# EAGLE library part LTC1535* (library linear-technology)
Isolated RS485 Transceiver Source : www.linear.com
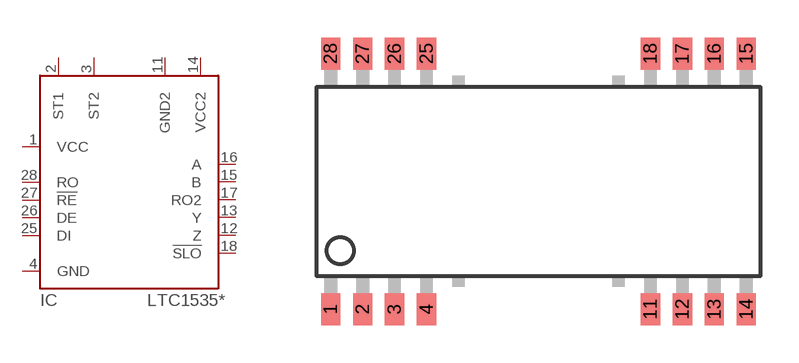
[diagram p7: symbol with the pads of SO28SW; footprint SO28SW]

Designator prefix IC

## LTC1535CSW (MPN: LTC1535CSW; OC_FARNELL: 1609802; OC_NEWARK: 56M1820), LTC1535ISW (MPN: LTC1535ISW; OC_FARNELL: 1498465; OC_NEWARK: 56M1824)  [SO28SW]
1  VCC  in
2  ST1  in
3  ST2  in
4  GND  in
11  GND2  in
12  Z  hiz
13  Y  hiz
14  VCC2  in
15  B  in
16  A  in
17  RO2  out
18  !SLO  in
25  DI  in
26  DE  in
27  !RE  in
28  RO  out

## Footprint SO28SW (pad centres in mm)
28-Lead Plastic Small Outline Isolation Barrier (Wide .300 Inch) Reference LTC DWG # 05-08-1690 Source: www.linear.com
smd 0.762 x 1.27: 1 -8.255,-5.08; 2 -6.985,-5.08; 3 -5.715,-5.08; 4 -4.445,-5.08; 11 4.445,-5.08; 12 5.715,-5.08; 13 6.985,-5.08; 14 8.255,-5.08; 15 8.255,5.08; 16 6.985,5.08; 17 5.715,5.08; 18 4.445,5.08; 25 -4.445,5.08; 26 -5.715,5.08; 27 -6.985,5.08; 28 -8.255,5.08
